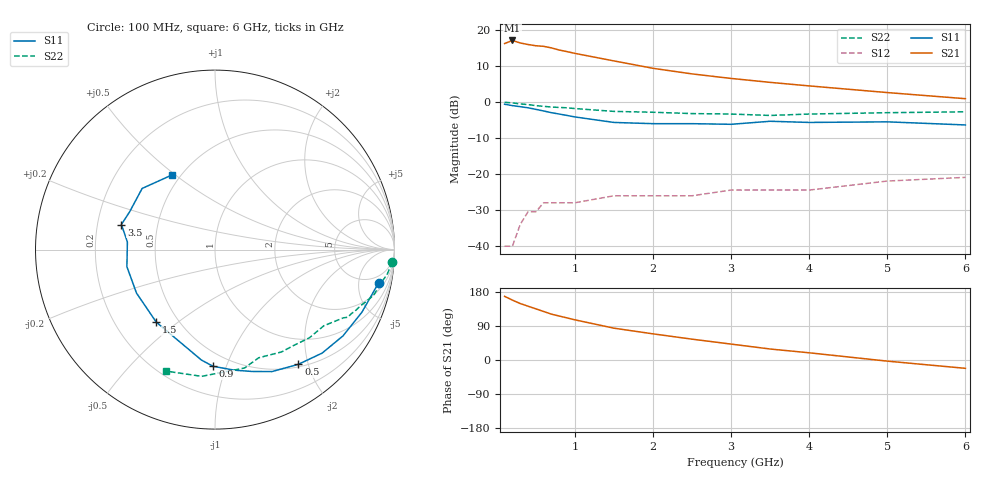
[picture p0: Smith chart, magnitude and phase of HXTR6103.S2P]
! HXTR-6103  (2N6618) Common Emitter
! Vce=10V  Ic=3mA
# ghz s ma r 50
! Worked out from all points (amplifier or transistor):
!   18 points, 100 MHz to 6 GHz, reference 50 ohm
!   highest |S21| = 17.1 dB at 200 MHz (marker M1)
!   |S21| within 3 dB of that: start of sweep to 877.4 MHz
!   unconditionally stable (mu >= 1): 1.7 GHz to end of sweep
!   at 400 MHz: K = 0.33, MSG = 23.2 dB, |S12| = -30.5 dB
!   at 1 GHz: K = 0.64, MSG = 20.7 dB, |S12| = -28.0 dB
!   at 6 GHz: K = 1.50, MAG = 6.7 dB, |S12| = -20.9 dB
!   S11 on the Smith chart (normalised r, x): 100 MHz: 3.20, -8.78; 500 MHz: 0.54, -1.84; 900 MHz: 0.40, -0.90; 1.5 GHz: 0.38, -0.42; 3.5 GHz: 0.30, +0.12; 6 GHz: 0.45, +0.49
0.1  0.93 -11.5  6.46 168.0  0.01 77.0  0.99 -4.0
0.2  0.89 -23.0  7.13 158.0  0.01 77.0  0.97 -8.0
0.3  0.86 -34.0  6.58 149.0  0.02 66.0  0.94 -12.0
0.4  0.83 -44.0  6.26 142.0  0.03 60.0  0.92 -16.0
0.5  0.79 -54.0  6.02 135.0  0.03 55.0  0.89 -19.0
0.6  0.75 -65.0  5.91 128.0  0.04 51.0  0.87 -21.0
0.7  0.71 -73.0  5.62 121.0  0.04 48.0  0.85 -24.0
0.8  0.68 -81.0  5.25 116.0  0.04 45.0  0.84 -25.0
0.9  0.65 -91.0  4.99 111.0  0.04 43.0  0.83 -27.0
1  0.62 -97.0  4.72 106.0  0.04 41.0  0.81 -28.0
1.5  0.52 -129.0  3.71 84.0  0.05 32.0  0.74 -35.0
2  0.5 -151.0  2.93 69.0  0.05 31.0  0.72 -43.0
2.5  0.5 -169.0  2.45 55.0  0.05 31.0  0.69 -51.0
3  0.49 175.0  2.12 42.0  0.06 33.0  0.68 -57.0
3.5  0.54 165.0  1.87 29.0  0.06 35.0  0.65 -68.0
4  0.52 156.0  1.67 19.0  0.06 37.0  0.68 -76.0
5  0.53 140.0  1.35 -3.0  0.08 35.0  0.71 -96.0
6  0.48 120.0  1.11 -22.0  0.09 34.0  0.73 -112.0
